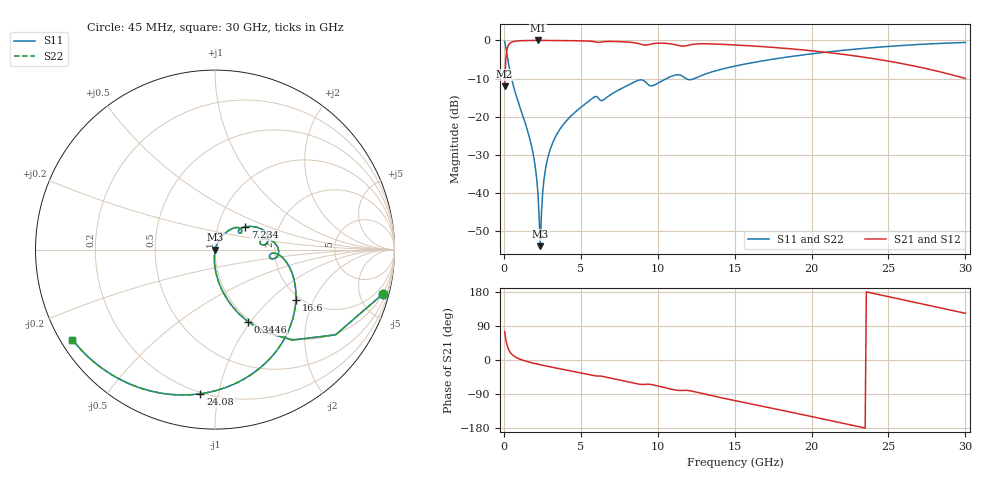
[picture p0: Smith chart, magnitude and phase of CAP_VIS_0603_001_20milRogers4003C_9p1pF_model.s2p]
! S-parameter model data by Modelithics Inc.  support@modelithics.com  813-866-6335  Tampa FL USA
! S-Parameter data specifications:
! Substrate: 20-mil Rogers 4003C, substrate thickness, H=0.508mm, Dielectric constant, Er=3.75
! PCB Mounting Pad Footprint: Pad width, PadW=0.90mm , Pad length, PadL=1.00mm , Pad gap, PadG (edge-to-edge)=1.00mm , Reference planes=3.0mm apart
! Created Wed Nov 18 13:25:29 2015
# hz S ma R 50
! 2 Port Network Data from SP1.SP block
! freq  magS11  angS11  magS21  angS21  magS12  angS12  magS22  angS22
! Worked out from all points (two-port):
!   401 points, 45 MHz to 30 GHz, reference 50 ohm
!   highest |S21| = -0.02 dB at 2.217 GHz (marker M1); lowest = -12.0 dB at 45 MHz (marker M2)
!   |S21| within 3 dB of the highest: 179.3 MHz to 20.71 GHz (20.54 GHz wide, 197 % of centre)
!   lowest |S11| = -53.9 dB at 2.367 GHz (marker M3), VSWR 1.00, Z = 50.2 - j0.00186 ohm
!   |S11| at or under -10 dB: 499 MHz to 10.56 GHz (10.06 GHz wide, 182 % of centre); 11.84 GHz to 12.39 GHz (545.9 MHz wide, 4.51 % of centre)
!   |S22| runs from -53.9 to -0.3 dB; largest |S21 - S12| = 0
!   S11 on the Smith chart (normalised r, x): 45 MHz: 0.97, -7.61; 344.6 MHz: 0.97, -0.97; 7.234 GHz: 1.35, +0.36; 16.6 GHz: 1.90, -1.47; 24.08 GHz: 0.19, -0.89; 30 GHz: 0.03, -0.29
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4.5e7  0.9681 -14.7  0.2504 75.3  0.2504 75.3  0.9681 -14.7
3.4455e8  0.4431 -65.4  0.8957 24.5  0.8957 24.5  0.4431 -65.4
7.189875e8  0.2146 -81.1  0.9756 8.6  0.9756 8.6  0.2146 -81.1
1.8423e9  0.03725 -95.0  0.9974 -7.6  0.9974 -7.6  0.03725 -95.0
2.066962e9  0.01992 -94.5  0.9978 -9.8  0.9978 -9.8  0.01992 -94.5
2.216738e9  0.009555 -89.7  0.9979 -11.2  0.9979 -11.2  0.009555 -89.7
2.366512e9  0.002018 -0.5  0.9978 -12.5  0.9978 -12.5  0.002018 -0.5
2.516288e9  0.009858 64.2  0.9977 -13.9  0.9977 -13.9  0.009858 64.2
2.74095e9  0.02275 68.8  0.9974 -15.8  0.9974 -15.8  0.02275 68.8
3.115388e9  0.04274 68.0  0.9965 -18.9  0.9965 -18.9  0.04274 68.0
3.864262e9  0.07921 63.1  0.9938 -25.0  0.9938 -25.0  0.07921 63.1
5.062462e9  0.1357 53.6  0.9859 -34.6  0.9859 -34.6  0.1357 53.6
7.2342e9  0.2113 36.9  0.9668 -50.4  0.9668 -50.4  0.2113 36.9
8.806838e9  0.3026 16.4  0.9024 -63.9  0.9024 -63.9  0.3026 16.4
1.007992e10  0.2807 12.5  0.9199 -69.4  0.9199 -69.4  0.2807 12.5
1.50225e10  0.4608 -19.0  0.8715 -107.2  0.8715 -107.2  0.4608 -19.0
1.659514e10  0.5297 -31.7  0.8341 -120.4  0.8341 -120.4  0.5297 -31.7
2.003996e10  0.668 -60.5  0.7301 -149.6  0.7301 -149.6  0.668 -60.5
2.408389e10  0.8071 -95.8  0.574 175.1  0.574 175.1  0.8071 -95.8
2.505742e10  0.8354 -104.4  0.5323 166.5  0.5323 166.5  0.8354 -104.4
2.737894e10  0.8929 -124.9  0.4303 146.0  0.4303 146.0  0.8929 -124.9
3e10  0.9398 -147.7  0.317 123.2  0.317 123.2  0.9398 -147.7
